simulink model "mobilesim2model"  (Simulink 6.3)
settings: Solver=ode3  StartTime=0.0  StopTime=100  FixedStep=dt  RelTol=1e-3
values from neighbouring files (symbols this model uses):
  D = 0.5    [mobilesim2demo.m]
  dt = 0.1    [mobilesim2demo.m]
  gmap = mobile1mapsim'    [mobilesim2demo.m]    (also in mobilesim2roadedge.m = reshape(inputs(4:end),4,81); mobile1mapsim.m = [mll,mrr])
  theta0 = x0    [mobilesim2demo.m]
  xy = [x0(:),y0(:)]    [mobilesim2demo.m]
libraries: simulink x2

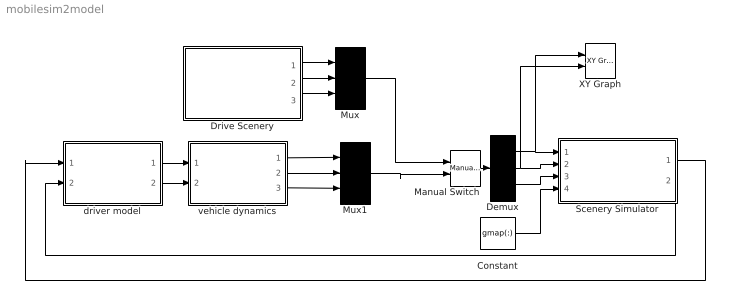
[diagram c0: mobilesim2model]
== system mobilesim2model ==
  Constant : Constant  Value=gmap(:)
  Demux : Demux  Outputs=3
  Drive Scenery : Subsystem
  Manual Switch : simulink/Signal Routing/Manual Switch  sw=0  action=0
  Mux : Mux  Inputs=3
  Mux1 : Mux  Inputs=3
  Scenery Simulator : Subsystem
  XY Graph : simulink/Sinks/XY Graph  xmin=0  xmax=100  ymin=0  ymax=100  st=-1
  driver model : Subsystem
  vehicle dynamics : Subsystem
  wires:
  driver model/2(steering) -> vehicle dynamics/2(steering1)
  Scenery Simulator/2(roadedge2) -> driver model/2(roadedge2)
  Scenery Simulator/1(roadedge) -> driver model/1(roadedge1)
  driver model/1(speed) -> vehicle dynamics/1(speed1)
  Demux/1 -> Scenery Simulator/1(xpos), XY Graph/1
  Demux/2 -> Scenery Simulator/2(ypos), XY Graph/2
  Demux/3 -> Scenery Simulator/3(theta)
  Manual Switch/1 -> Demux/1
  vehicle dynamics/1(xpos) -> Mux1/1
  vehicle dynamics/2(ypos) -> Mux1/2
  vehicle dynamics/3(theta) -> Mux1/3
  Mux1/1 -> Manual Switch/2
  Mux/1 -> Manual Switch/1
  Drive Scenery/3(theta) -> Mux/3
  Drive Scenery/2(y-position) -> Mux/2
  Drive Scenery/1(x-position) -> Mux/1
  Constant/1 -> Scenery Simulator/4(gmap)

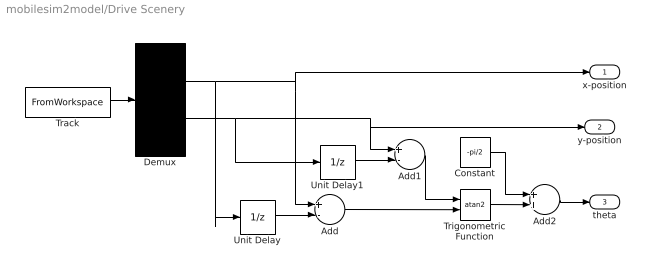
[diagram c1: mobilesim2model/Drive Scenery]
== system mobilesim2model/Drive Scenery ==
  Add : Sum  Inputs=+-  OutScaling=2^-10
  Add1 : Sum  Inputs=+-  OutScaling=2^-10
  Add2 : Sum  OutScaling=2^-10
  Constant : Constant  Value=-pi/2
  Demux : Demux  Outputs=2
  Track : FromWorkspace  VariableName=[t,xy]  SampleTime=dt
  Trigonometric Function : Trigonometry  Operator=atan2
  Unit Delay : UnitDelay  SampleTime=-1
  Unit Delay1 : UnitDelay  SampleTime=-1
  x-position : Outport
  y-position : Outport  Port=2
  theta : Outport  Port=3
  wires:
  Demux/2 -> Unit Delay1/1, y-position/1, Add1/1
  Demux/1 -> Unit Delay/1, Add/1, x-position/1
  Track/1 -> Demux/1
  Unit Delay/1 -> Add/2
  Add2/1 -> theta/1
  Constant/1 -> Add2/1
  Trigonometric Function/1 -> Add2/2
  Add/1 -> Trigonometric Function/2
  Add1/1 -> Trigonometric Function/1
  Unit Delay1/1 -> Add1/2

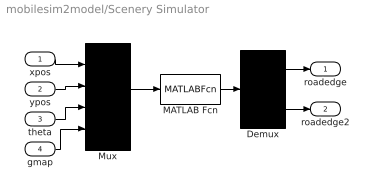
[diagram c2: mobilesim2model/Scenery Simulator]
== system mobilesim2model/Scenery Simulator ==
  xpos : Inport
  ypos : Inport  Port=2
  theta : Inport  Port=3
  gmap : Inport  Port=4
  Demux : Demux  Outputs=2
  MATLAB Fcn : MATLABFcn  MATLABFcn=mobilesim2roadedge
  Mux : Mux
  roadedge : Outport
  roadedge2 : Outport  Port=2
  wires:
  Mux/1 -> MATLAB Fcn/1
  MATLAB Fcn/1 -> Demux/1
  Demux/1 -> roadedge/1
  xpos/1 -> Mux/1
  ypos/1 -> Mux/2
  Demux/2 -> roadedge2/1
  theta/1 -> Mux/3
  gmap/1 -> Mux/4

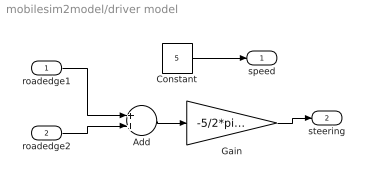
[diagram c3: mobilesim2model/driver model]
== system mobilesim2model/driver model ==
  roadedge1 : Inport
  roadedge2 : Inport  Port=2
  Add : Sum  OutScaling=2^-10
  Constant : Constant  Value=5
  Gain : Gain  Gain=-5/2*pi/180
  speed : Outport
  steering : Outport  Port=2
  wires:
  Constant/1 -> speed/1
  Gain/1 -> steering/1
  Add/1 -> Gain/1
  roadedge1/1 -> Add/1
  roadedge2/1 -> Add/2

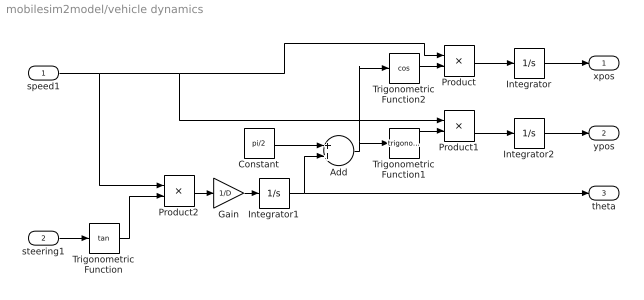
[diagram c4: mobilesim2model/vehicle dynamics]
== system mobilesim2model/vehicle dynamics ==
  speed1 : Inport
  steering1 : Inport  Port=2
  Add : Sum  OutScaling=2^-10
  Constant : Constant  Value=pi/2
  Gain : Gain  Gain=1/D
  Integrator : Integrator  InitialCondition=xy(1,1)
  Integrator1 : Integrator  InitialCondition=theta0(1)
  Integrator2 : Integrator  InitialCondition=xy(1,2)
  Product : Product
  Product1 : Product
  Product2 : Product
  Trigonometric Function : Trigonometry  Operator=tan
  Trigonometric Function1 : Trigonometry
  Trigonometric Function2 : Trigonometry  Operator=cos
  xpos : Outport
  ypos : Outport  Port=2
  theta : Outport  Port=3
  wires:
  speed1/1 -> Product/1, Product1/1, Product2/1
  steering1/1 -> Trigonometric Function/1
  Gain/1 -> Integrator1/1
  Trigonometric Function1/1 -> Product1/2
  Product1/1 -> Integrator2/1
  Product/1 -> Integrator/1
  Integrator/1 -> xpos/1
  Integrator2/1 -> ypos/1
  Integrator1/1 -> theta/1, Add/2
  Trigonometric Function2/1 -> Product/2
  Trigonometric Function/1 -> Product2/2
  Product2/1 -> Gain/1
  Constant/1 -> Add/1
  Add/1 -> Trigonometric Function1/1, Trigonometric Function2/1
